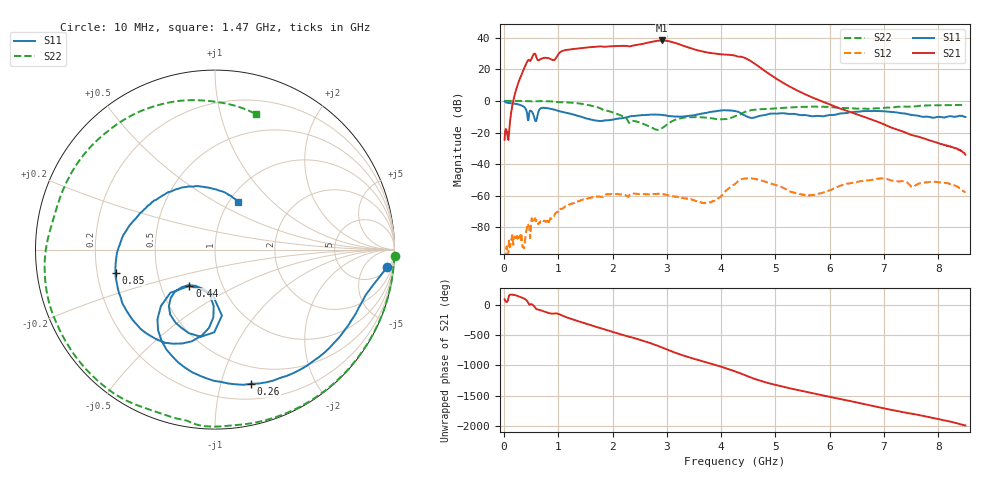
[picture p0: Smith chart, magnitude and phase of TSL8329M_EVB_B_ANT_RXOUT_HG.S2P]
!Agilent Technologies,E5071C,MY46523237,B.13.01
!Date: Tue Aug 02 11:43:03 2022
!Data & Calibration Information:
!Freq	S11:SOLT2(ON)	S21:SOLT2(ON)	S12:SOLT2(ON)	S22:SOLT2(ON)
!PortZ  Port1:50+j0  Port2:50+j0
!Above PortZ is port z conversion or system Z0 setting when saving the data.
!When reading, reference impedance value at option line is always used.
# Hz S dB R 50
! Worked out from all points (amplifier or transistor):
!   850 points, 10 MHz to 8.5 GHz, reference 50 ohm
!   highest |S21| = 38.2 dB at 2.91 GHz (marker M1)
!   |S21| within 3 dB of that: 2.415 GHz to 3.275 GHz (859.8 MHz wide, 30.2 % of centre)
!   unconditionally stable (mu >= 1): 14.96 MHz to end of sweep
!   at 1.42 GHz: K = 4.69, MAG = 38.3 dB, |S12| = -62.7 dB
!   at 4.26 GHz: K = 5.24, MAG = 30.3 dB, |S12| = -52.4 dB
!   at 8.5 GHz: K = 7208.13, MAG = -30.0 dB, |S12| = -57.2 dB
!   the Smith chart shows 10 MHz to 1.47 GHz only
!   S11 on the Smith chart (normalised r, x): 10 MHz: 6, -18; 260 MHz: 0.33, -1.25; 440 MHz: 0.70, -0.30; 850 MHz: 0.28, -0.11; 1.47 GHz: 1.10, +0.64
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1e7  -0.31 -5.7  -24.57 90.9  -97.77 -169.8  0.01 -2.0
2.6e8  -2.23 -75.0  11.18 142.6  -86.36 44.6  -0.03 -52.0
4.4e8  -12.14 -125.1  25.65 43.1  -77.99 73.5  -0.13 -87.4
6e8  -11.67 -96.0  27.17 -71.3  -75.26 38.3  -0.28 -116.2
8.5e8  -4.90 -167.0  26.55 -141.2  -74.24 42.3  -0.28 -164.3
1.13e9  -7.42 137.3  32.09 161.5  -66.70 10.1  -0.89 144.1
1.43e9  -10.13 73.2  33.31 71.9  -62.64 -38.4  -1.84 81.8
1.47e9  -10.58 64.3  33.51 60.7  -62.25 -44.4  -2.06 73.1
1.73e9  -12.63 -6.5  34.33 -13.0  -60.52 -88.8  -4.13 11.4
2e9  -11.86 -79.1  34.57 -86.2  -58.95 -130.1  -7.28 -53.1
2.42e9  -9.42 -161.5  35.22 165.1  -58.70 172.0  -12.87 -148.9
2.68e9  -8.72 154.9  37.02 93.0  -59.05 139.0  -16.15 135.8
2.84e9  -8.65 125.9  38.06 40.4  -58.66 116.7  -18.30 53.2
2.91e9  -8.88 112.2  38.19 15.4  -58.77 106.3  -17.30 9.1
3.14e9  -9.83 73.3  36.80 -65.9  -60.45 77.5  -12.11 -88.5
3.44e9  -9.34 23.1  33.26 -154.9  -62.07 50.0  -10.28 -154.6
3.84e9  -6.75 -51.1  30.05 101.6  -63.56 53.5  -11.06 152.2
4.26e9  -6.48 -126.7  28.57 -20.8  -52.41 20.7  -9.59 118.9
4.62e9  -10.40 -149.2  23.49 -143.3  -49.28 -78.8  -5.54 40.6
5.67e9  -9.72 65.9  2.31 -16.0  -59.63 27.2  -3.64 -144.7
7.09e9  -6.84 -174.8  -16.19 74.2  -49.84 123.9  -4.29 -26.2
8.5e9  -10.16 -88.0  -34.01 169.0  -57.24 -33.5  -2.49 124.0
